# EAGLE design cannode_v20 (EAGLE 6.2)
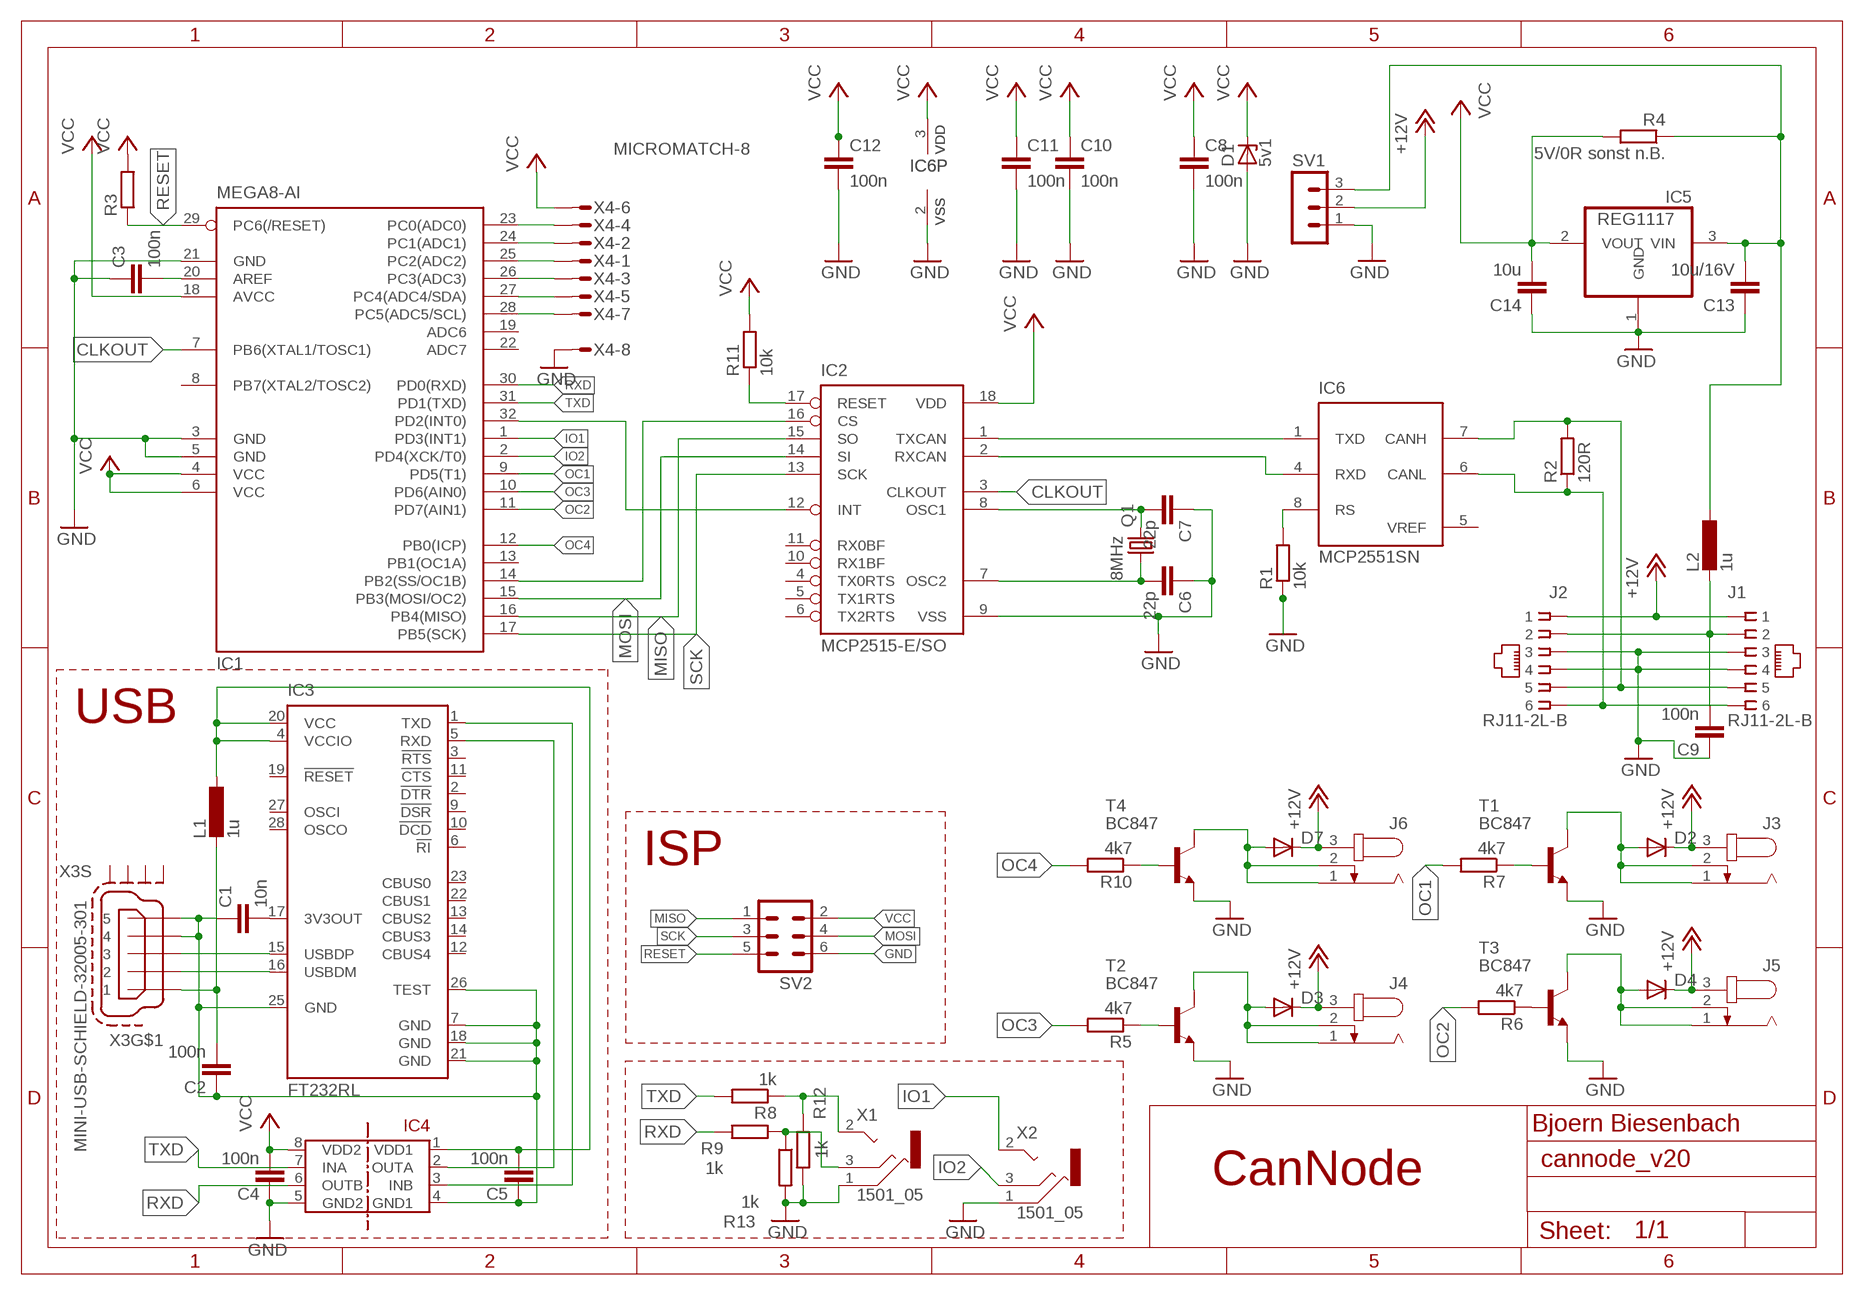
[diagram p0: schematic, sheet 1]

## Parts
C1  10n  C0805  [0805]
C2  100n  C0805  [0805]
C3  100n  C0805  [0805]
C4  100n  C0805  [0805]
C5  100n  C0805  [0805]
C6  22p  C0805  [0805]
C7  22p  C0805  [0805]
C8  100n  C0805  [0805]
C9  100n  C0805  [0805]
C10  100n  C0805  [0805]
C11  100n  C0805  [0805]
C12  100n  C0805  [0805]
C13  10u/16V  C0805  [0805]
C14  10u  C0805  [0805]
D1  5v1  ZENER-DIODESOD80C  [SOD80C]
D2  DIODE-MINIMELF  [MINIMELF]
D3  DIODE-MINIMELF  [MINIMELF]
D4  DIODE-MINIMELF  [MINIMELF]
D7  DIODE-MINIMELF  [MINIMELF]
IC1  MEGA8-AI  [TQFP32-08]
IC2  MCP2515-E/SO  [SO18L]
IC3  FT232RL  [SSOP28]
IC4  ADUM1201  [SO8]
IC5  REG1117  [SOT223]
IC6  MCP2551SN  [SO-08]
J1  RJ11-2L-B  [RJ11-NO_SHIELD]
J2  RJ11-2L-B  [RJ11-NO_SHIELD]
J3  JACK-PLUG0  [SPC4077]
J4  JACK-PLUG0  [SPC4077]
J5  JACK-PLUG0  [SPC4077]
J6  JACK-PLUG0  [SPC4077]
L1  1u  L0805  [0805]
L2  1u  L0805  [0805]
Q1  8MHz  CRYSTALHC49U70  [HC49U70]
R1  10k  R0805  [0805]
R2  120R  R0805  [0805]
R3  R0805  [0805]
R4  5V/0R sonst n.B.  R0805  [0805]
R5  4k7  R0805  [0805]
R6  4k7  R0805  [0805]
R7  4k7  R0805  [0805]
R8  1k  R0805  [0805]
R9  1k  R0805  [0805]
R10  4k7  R0805  [0805]
R11  10k  R0805  [0805]
R12  1k  R0805  [0805]
R13  1k  R0805  [0805]
SV1  MA03-1  [MA03-1]
SV2  MA03-2  [MA03-2]
T1  BC847  [SOT23]
T2  BC847  [SOT23]
T3  BC847  [SOT23]
T4  BC847  [SOT23]
X1  1501_05  [1501_05]
X2  1501_05  [1501_05]
X3  MINI-USB-SCHIELD-32005-301  [32005-301]
X4  MICROMATCH-8  [MICROMATCH-8]

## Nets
+12V: D2.C D3.C D4.C D7.C J1.1 J2.1 J3.3 J4.3 J5.3 J6.3 SV1.2
CLKOUT: IC1.7(PB6(XTAL1/TOSC1)) IC2.3(CLKOUT)
GND: C3.1 C4.1 C6.1 C7.1 C8.2 C9.1 C10.2 C11.2 C12.2 C13.1 C14.1 D1.A IC1.3(GND) IC1.5(GND) IC1.21(GND) IC2.9(VSS) IC4.5(GND2) IC5.1(GND) IC6.2(VSS) J1.3 J1.4 J2.3 J2.4 R1.1 R12.2 R13.2 SV1.1 SV2.6 T1.2(E) T2.2(E) T3.2(E) T4.2(E) X1.1 X2.1 X4.8
GND_USB: C1.1 C2.1 C5.1 IC3.7(GND) IC3.18(GND) IC3.21(GND) IC3.25(GND) IC3.26(TEST) IC4.4(GND1) X3.4 X3.5
IO1: IC1.1(PD3(INT1)) X2.2
IO2: IC1.2(PD4(XCK/T0)) X2.3
MISO: IC1.16(PB4(MISO)) IC2.15(SO) SV2.1
MOSI: IC1.15(PB3(MOSI/OC2)) IC2.14(SI) SV2.4
N$1: C7.2 IC2.8(OSC1) Q1.2
N$2: C6.2 IC2.7(OSC2) Q1.1
N$3: IC2.1(TXCAN) IC6.1(TXD)
N$4: IC2.2(RXCAN) IC6.4(RXD)
N$5: IC6.7(CANH) J1.5 J2.5 R2.2
N$6: IC6.6(CANL) J1.6 J2.6 R2.1
N$7: IC6.8(RS) R1.2
N$8: IC1.14(PB2(SS/OC1B)) IC2.16(CS)
N$9: IC1.32(PD2(INT0)) IC2.12(INT)
N$10: C3.2 IC1.20(AREF)
N$11: IC2.17(RESET) R11.1
N$12: IC3.15(USBDP) X3.3
N$13: IC3.16(USBDM) X3.2
N$14: C5.2 IC3.4(VCCIO) IC3.20(VCC) IC4.1(VDD1) L1.1
N$15: R9.1 R13.1 X1.3
N$16: C9.2 J1.2 J2.2 L2.2
N$17: C2.2 L1.2 X3.1
N$18: C13.2 IC5.3(VIN) L2.1 R4.1 SV1.3
N$20: C1.2 IC3.17(3V3OUT)
N$21: R6.1 T3.1(B)
N$22: D4.A J5.1 J5.2 T3.3(C)
N$24: R5.1 T2.1(B)
N$25: R7.1 T1.1(B)
N$26: IC3.5(RXD) IC4.2(OUTA)
N$27: D2.A J3.1 J3.2 T1.3(C)
N$28: D3.A J4.1 J4.2 T2.3(C)
N$29: IC3.1(TXD) IC4.3(INB)
N$30: R8.1 R12.1 X1.2
N$31: D7.A J6.1 J6.2 T4.3(C)
N$32: IC1.28(PC5(ADC5/SCL)) X4.7
N$33: IC1.27(PC4(ADC4/SDA)) X4.5
N$34: R10.1 T4.1(B)
N$35: IC1.26(PC3(ADC3)) X4.3
N$36: IC1.25(PC2(ADC2)) X4.1
N$37: IC1.24(PC1(ADC1)) X4.2
N$38: IC1.23(PC0(ADC0)) X4.4
OC1: IC1.9(PD5(T1)) R7.2
OC2: IC1.11(PD7(AIN1)) R6.2
OC3: IC1.10(PD6(AIN0)) R5.2
OC4: IC1.12(PB0(ICP)) R10.2
RESET: IC1.29(PC6(/RESET)) R3.1 SV2.5
RXD: IC1.30(PD0(RXD)) IC4.6(OUTB) R9.2
SCK: IC1.17(PB5(SCK)) IC2.13(SCK) SV2.3
TXD: IC1.31(PD1(TXD)) IC4.7(INA) R8.2
VCC: C4.2 C8.1 C10.1 C11.1 C12.1 C14.2 D1.C IC1.4(VCC) IC1.6(VCC) IC1.18(AVCC) IC2.18(VDD) IC4.8(VDD2) IC5.2(VOUT) IC6.3(VDD) R3.2 R4.2 R11.2 SV2.2 X4.6
Unconnected: IC1.8(PB7(XTAL2/TOSC2)) IC1.13(PB1(OC1A)) IC1.19(ADC6) IC1.22(ADC7) IC2.4(TX0RTS) IC2.5(TX1RTS) IC2.6(TX2RTS) IC2.10(RX1BF) IC2.11(RX0BF) IC3.2(!DTR) IC3.3(!RTS) IC3.6(!RI) IC3.9(!DSR) IC3.10(!DCD) IC3.11(!CTS) IC3.12(CBUS4) IC3.13(CBUS2) IC3.14(CBUS3) IC3.19(!RESET) IC3.22(CBUS1) IC3.23(CBUS0) IC3.27(OSCI) IC3.28(OSCO) X3.M1(S:S1) X3.M2(S:S2) X3.M3(S:S3) X3.M4(S:S4)

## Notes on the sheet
- USB
- ISP
- Bjoern Biesenbach
- CanNode

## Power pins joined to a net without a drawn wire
VREF: IC6.5(VREF)

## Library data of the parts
C1-C14 = R_C_0805:C0805
D1 = diode:ZENER-DIODE: Z-Diode
D2-D4 D7 = diode:DIODE-: DIODE
IC1 = atmel:MEGA8: MICROCONTROLLER 8 Kbytes FLASH, 1 kbytes SRAM, 512 bytes EEPROM, USART, 6-channel 10 bit ADC, 2-channel 8 bit ADC Pin compatible with Atmega48, ATMega88, ATMega168 Source: avr.lbr; MPN: ATMEGA8-16AU; OC_FARNELL: 9171371; OC_NEWARK: 73M8863
IC2 = mcp2515:MCP2515
IC3 = ftdichip:FT232R: Source: http://www.ftdichip.com/Documents/DataSheets/DS_FT232R_v104.pdf; MPN: FT232RL; OC_FARNELL: 1146032; OC_NEWARK: 91K9918
IC4 = Bus-isolators:ADUM1201
IC5 = burr-brown:REG1117: 800mA and 1A Low Dropout (LDO) Positive Regulator 1.8V, 2.5V, 2.85V, 3.3V, 5V, and Adj; MPN: REG1117; OC_FARNELL: 1097566; OC_NEWARK: 14P6981
IC6 = microchip_can:MCP2551: High Speed CAN tranceiver
J1 J2 = con-tycoelectronics:RJ11: CORCOM Modular RJ Jacks No Shield Source: www.tycoelectronics.com .. ENG_DS_1654001_1099_RJ_L_0507.pdf; MF: TYCO ELECTRONICS; MPN: RJ11-2L-B; OC_FARNELL: unknown; OC_NEWARK: 83F4463
J3-J6 = con-jack:JACK-PLUG: DC POWER JACK Power Jack, DC, Right Angle, Through Hole, Rated 5A at 16VDC, PC Terminals Distributor: Farnell (www.Farnell.de) Drawing: 84N1161.pdf / 84N1162.pdf Manufacturer: SPC Technology (www.spctechnology.com) Type: SPC4077 / SPC 4078; OC_FARNELL: unknown; OC_NEWARK: unknown
L1 L2 = R_C_0805:L0805
Q1 = crystal:CRYSTAL: CRYSTAL; OC_FARNELL: unknown; OC_NEWARK: unknown
R1-R13 = R_C_0805:R0805
SV1 = con-lstb:MA03-1: PIN HEADER; OC_FARNELL: unknown; OC_NEWARK: unknown
SV2 = con-lstb:MA03-2: PIN HEADER; OC_FARNELL: unknown; OC_NEWARK: unknown
T1-T4 = transistor:BC847: NPN TRANSISTOR
X1 X2 = con-lumberg:1501_0*: Jack connectors according to JISC 6560, 2.5 mm Klinkensteckverbinder nach JISC 6560, 2,5 mm Source: http://www.lumberg.com/Produkte/PDFs/1501_05.pdfedit 1501_03 http://www.lumberg.com/Produkte/PDFs/1501_06.pdf; OC_FARNELL: 1216978; OC_NEWARK: unknown
X3 = con-cypressindustries:MINI-USB-SCHIELD-: MINI USB-B Conector Source: www.cypressindustries.com; OC_FARNELL: unknown; OC_NEWARK: unknown
X4 = con-amp-micromatch:MICROMATCH-8: MicroMaTch 8 7-215464-8 / 0-215464-8 Drawing Number C-215464 DDEController.pdf; MF: FARNELL; MPN: 7-215464-8; OC_FARNELL: 3784642; OC_NEWARK: 26H0301

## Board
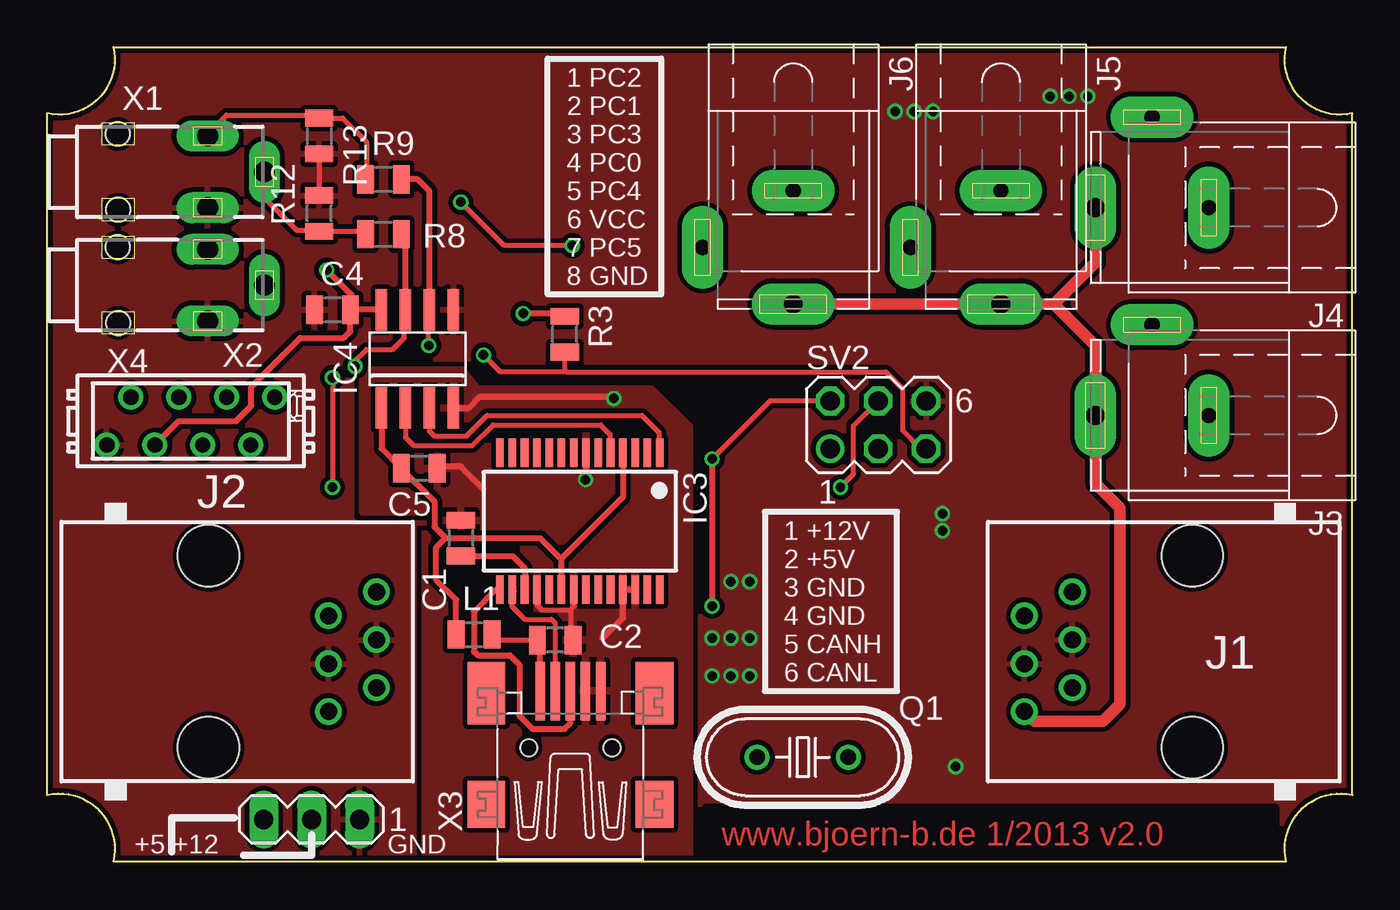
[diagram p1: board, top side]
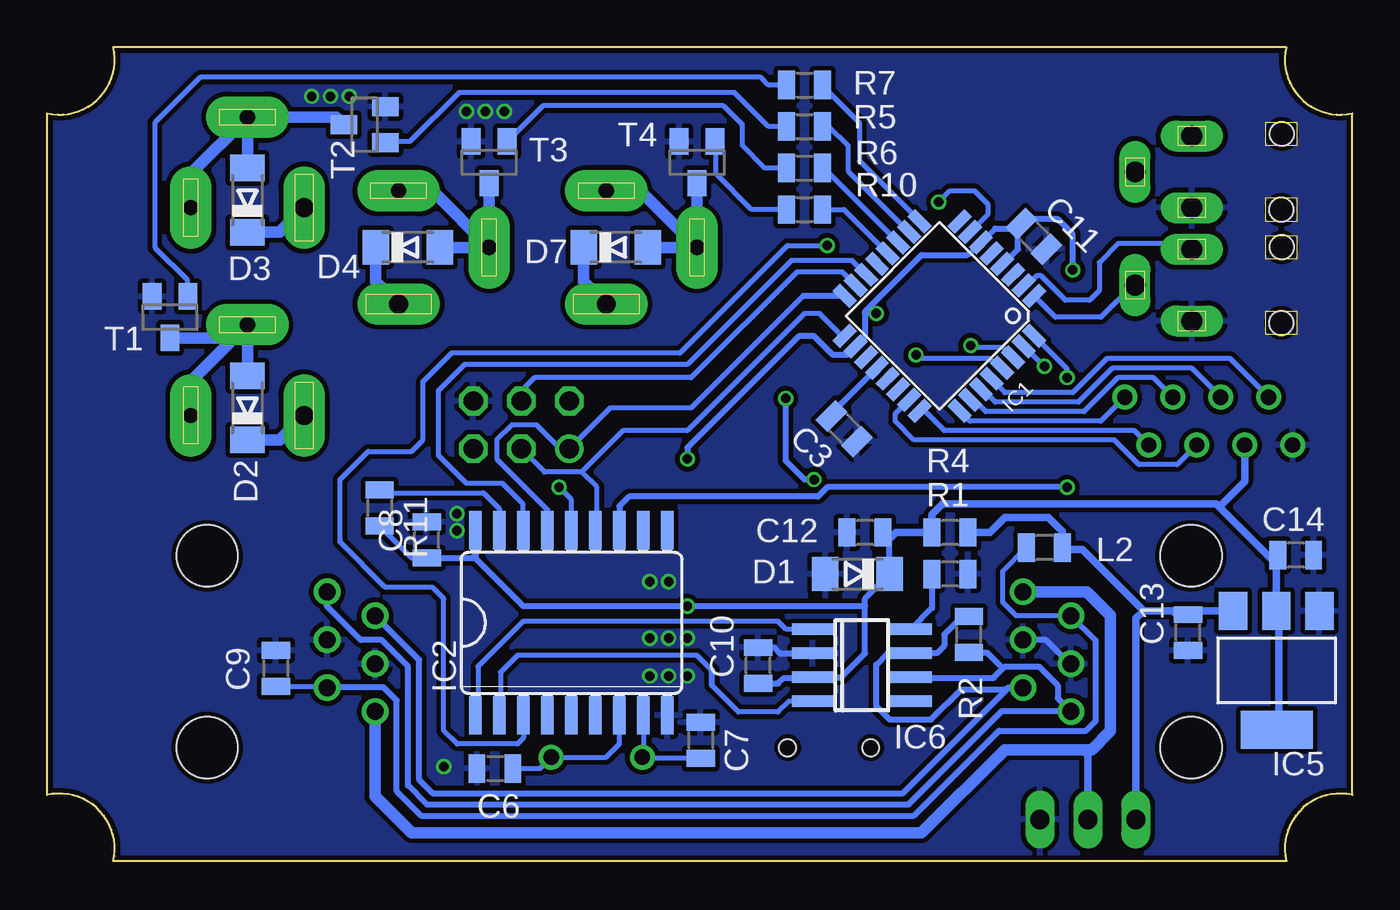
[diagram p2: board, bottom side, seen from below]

Size 69.1 x 43.1 mm. Coordinates in mm from the lower left corner, seen from the top.
Outline: 3.5,0 65.6,0 arc-116 69.1,3.5 69.1,39.6 arc-116 65.6,43.1 3.5,43.1 arc-116 0,39.6 0,3.5 arc-116 3.5,0
Copper layers (1*16): Top 0.035mm / dielectric 1.5mm / Bottom 0.035mm
Design rules: minimum track width 6mil, minimum drill 12mil, track to track 6mil, track to pad 6mil, pad to pad 6mil, via to via 6mil, smd to smd 0mil, copper to edge 10mil, drill to drill 10mil, minimum pad ring 10mil, minimum via ring 6mil, stop-mask expansion 2mil, vias tented up to drill 100mil, thermal gap 10mil
tRestrict: area 34.9,0 to 65,2.8

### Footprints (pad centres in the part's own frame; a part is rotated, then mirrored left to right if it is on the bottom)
0805 = smd 0.894 x 1.5: 1 -0.95,0; 2 0.95,0
SOD80C = smd 1.4 x 1.8: A 1.7,0; C -1.7,0
MINIMELF = smd 1.4 x 1.8: A 1.7,0; C -1.7,0
TQFP32-08 = smd 1.27 x 0.559: 1 -4.293,2.8; 2 -4.293,2; 3 -4.293,1.2; 4 -4.293,0.4; 5 -4.293,-0.4; 6 -4.293,-1.2; 7 -4.293,-2; 8 -4.293,-2.8; 17 4.293,-2.8; 18 4.293,-2; 19 4.293,-1.2; 20 4.293,-0.4; 21 4.293,0.4; 22 4.293,1.2; 23 4.293,2; 24 4.293,2.8 | smd 0.559 x 1.27: 9 -2.8,-4.293; 10 -2,-4.293; 11 -1.2,-4.293; 12 -0.4,-4.293; 13 0.4,-4.293; 14 1.2,-4.293; 15 2,-4.293; 16 2.8,-4.293; 25 2.8,4.293; 26 2,4.293; 27 1.2,4.293; 28 0.4,4.293; 29 -0.4,4.293; 30 -1.2,4.293; 31 -2,4.293; 32 -2.8,4.293
SO18L = smd 0.66 x 2.032: 1 -5.08,-4.902; 2 -3.81,-4.902; 3 -2.54,-4.902; 4 -1.27,-4.902; 5 0,-4.902; 6 1.27,-4.902; 7 2.54,-4.902; 8 3.81,-4.902; 9 5.08,-4.902; 10 5.08,4.902; 11 3.81,4.902; 12 2.54,4.902; 13 1.27,4.902; 14 0,4.902; 15 -1.27,4.902; 16 -2.54,4.902; 17 -3.81,4.902; 18 -5.08,4.902
SSOP28 = smd 0.4 x 1.5: 1 -4.225,-3.625; 2 -3.575,-3.625; 3 -2.925,-3.625; 4 -2.275,-3.625; 5 -1.625,-3.625; 6 -0.975,-3.625; 7 -0.325,-3.625; 8 0.325,-3.625; 9 0.975,-3.625; 10 1.625,-3.625; 11 2.275,-3.625; 12 2.925,-3.625; 13 3.575,-3.625; 14 4.225,-3.625; 15 4.225,3.625; 16 3.575,3.625; 17 2.925,3.625; 18 2.275,3.625; 19 1.625,3.625; 20 0.975,3.625; 21 0.325,3.625; 22 -0.325,3.625; 23 -0.975,3.625; 24 -1.625,3.625; 25 -2.275,3.625; 26 -2.925,3.625; 27 -3.575,3.625; 28 -4.225,3.625
SO8 = smd 0.6 x 2.2: 1 -1.905,-2.6; 2 -0.635,-2.6; 3 0.635,-2.6; 4 1.905,-2.6; 5 1.905,2.6; 6 0.635,2.6; 7 -0.635,2.6; 8 -1.905,2.6
SOT223 = smd 1.499 x 2.007: 1 -2.261,-3.15; 2 0.025,-3.15; 3 2.311,-3.15 | smd 3.81 x 2.007: 4 0,3.15
SO-08 = smd 0.6 x 2.2: 1 -1.905,-2.6; 2 -0.635,-2.6; 3 0.635,-2.6; 4 1.905,-2.6; 5 1.905,2.6; 6 0.635,2.6; 7 -0.635,2.6; 8 -1.905,2.6
RJ11-NO_SHIELD = drill 0.9 pad 1.4: 1 -3.175,8.89; 2 -1.905,6.35; 3 -0.635,8.89; 4 0.635,6.35; 5 1.905,8.89; 6 3.175,6.35 | hole 3.251: -5.08,0; 5.08,0
SPC4077 = drill 0.8 pad 2.184 long: 1 -3,0; 2 0,-4.8 | drill 1 pad 2.184 long: 3 3,0
HC49U70 = drill 0.813: 1 -2.413,0; 2 2.413,0
MA03-1 = drill 1.016 long: 1 -2.54,0; 2 0,0; 3 2.54,0
MA03-2 = drill 1.016: 1 -2.54,-1.27 | drill 1.016 octagon: 2 -2.54,1.27; 3 0,-1.27; 4 0,1.27; 5 2.54,-1.27; 6 2.54,1.27
SOT23 = smd 1 x 1.4: 1 -0.95,-1.1; 2 0.95,-1.1; 3 0,1.1
1501_05 = drill 1.1 pad 1.4 long: 1 -1.9,-8.5; 2 0,-11.5; 3 1.9,-8.5 | hole 1.27: -2.007,-3.759; 2.007,-3.734
32005-301 = smd 3.1 x 0.5: 1 3,1.6; 2 3,0.8; 3 3,0; 4 3,-0.8; 5 3,-1.6 | smd 2.5 x 2: M1 -3,-4.45; M2 -3,4.45 | smd 3.3 x 2: M3 2.9,4.45; M4 2.9,-4.45 | hole 0.9: 0,2.2; 0,-2.2
MICROMATCH-8 = drill 0.813: 1 4.445,1.27; 2 3.175,-1.27; 3 1.905,1.27; 4 0.635,-1.27; 5 -0.635,1.27; 6 -1.905,-1.27; 7 -3.175,1.27; 8 -4.445,-1.27

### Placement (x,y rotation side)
C1  21.9,17.1 270 top
C2  26.9,11.7 180 top
C3  26.9,22.9 135 bottom
C4  15.1,29.2 0 top
C5  19.7,20.8 180 top
C6  45.4,4.9 0 bottom
C7  34.5,6.4 270 bottom
C8  49,17 90 bottom
C9  57,10.2 270 bottom
C10  31.46,10.35 90 bottom
C11  16.86,33.08 315 bottom
C12  25.8,17.4 180 bottom
C13  8.7,12.1 90 bottom
C14  3,16.2 180 bottom
D1  26.2,15.2 180 bottom
D2  58.5,24 90 bottom
D3  58.5,35 90 bottom
D4  50,32.5 0 bottom
D7  39,32.5 0 bottom
IC1  21.85,28.87 225 bottom
IC2  41.34,12.62 0 bottom
IC3  28.2,18 180 top
IC4  19.6,26.6 0 top
IC5  4,10.1 180 bottom
IC6  25.97,10.37 270 bottom
J1  60.63,11.09 90 top
J2  8.54,11.09 270 top
J3  58.5,23.6 180 top
J4  58.5,34.6 180 top
J5  50.5,32.5 270 top
J6  39.5,32.5 270 top
L1  22.6,12 0 top
L2  16.3,16.6 180 bottom
Q1  40,5.5 180 top
R1  21.3,15.2 180 bottom
R2  20.3,12 90 bottom
R3  27.4,27.9 90 top
R4  21.3,17.4 180 bottom
R5  29,38.9 0 bottom
R6  29,36.7 0 bottom
R7  29,41.1 0 bottom
R8  17.8,33.2 0 top
R9  17.8,36.1 0 top
R10  29,34.5 0 bottom
R11  51.5,18.7 270 bottom
R12  14.4,34.3 90 top
R13  14.4,38.4 270 top
SV1  14,2.2 180 top
SV2  44,23.1 0 top
T1  62.6,28.8 180 bottom
T2  52.3,39 90 bottom
T3  45.7,37 180 bottom
T4  34.7,37 180 bottom
X1  0,36.5 90 top
X2  0,30.5 90 top
X3  27.7,6 90 top
X4  7.6,23.3 0 top

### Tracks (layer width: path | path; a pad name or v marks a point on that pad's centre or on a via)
+12V
  Top 0.61: J1.1 52.26,7.4 55.9,7.4 56.8,8.3 56.8,18.7 55.5,20 J3.3 55.5,27.3 53.3,29.5 | 53.3,29.5 J5.3 J6.3 | J4.3 55.5,31.7 53.3,29.5
  Bottom 0.4: SV1.2 14,5.6 14.3,5.9
  Bottom 0.61: J2.1 14.06,14.27 12.8,13 12.8,6.9 13.8,5.9 14.3,5.9 18.4,5.9 22.8,1.5 49.8,1.5 51.74,3.44 J1.1 | J3.3 56.8,22.3 D2.C | D3.C 56.8,33.3 J4.3 | D4.C 51.7,30.7 J5.3 | D7.C 40.7,30.7 J6.3
CLKOUT  (via drill 0.5)
  Top 0.254: v27.8,32.6 24.2,32.6 v21.9,34.9
  Bottom 0.254: IC1.7 19.3,34.25 19.3,34.8 20,35.5 21.3,35.5 v21.9,34.9 | v27.8,32.6 29.9,32.6 35.6,26.9 47.7,26.9 49.2,25.4 49.2,22.3 49.8,21.7 52.1,21.7 53.6,20.2 53.6,16.9 51.2,14.5 48.7,14.5 48.1,13.9 48.1,6.9 47.4,6.2 44.2,6.2 43.88,6.52 IC2.3
GND  (via drill 0.5)
  Top 0.254: R13.2 R12.2
  Bottom 0.305: C10.2 30.6,11.3 30.3,11 IC6.2 | J2.4 14.96,10.46 16.23,11.72 J2.3
  other vias: 44.9,39.7 45.9,39.7 46.9,39.7 53.1,40.5 54.1,40.5 55.1,40.5 47.4,18.4 37.2,11.8 36.2,11.8 35.2,11.8 35.2,9.8 36.2,9.8 37.2,9.8 48.1,5 47.4,17.5 37.2,14.8 36.2,14.8
  pour Bottom (isolate 0.254): 0,0 69,0 69,43 69,43.5 0,43.5
  pour Top (isolate 0.254, rank 2): 0,0 69.5,0 69.5,43 69.5,43.5 0,43.5
GND_USB  (via drill 0.5)
  Top 0.254: IC3.18 25.93,13.57 26.2,13.3 27.7,13.3 | 27.7,13.3 27.9,13.5 27.9,14.35 IC3.21 | 27.7,13.3 27.7,11.95 C2.1
  Top 0.305: IC3.26 IC3.25 30.5,14.35 30.5,12.9 29.4,11.8 | IC3.7 28.52,20.38 28.6,20.3 | IC4.4 22.3,24 22.9,24.6 29.9,24.6 v30,24.5 | 23.1,19.7 21.9,20.9 20.9,20.9 20.7,20.7 20.6,20.7
  Bottom 0.305: v30,24.5 30,21.2 29,20.2 v28.5,20.2
  pour Top (isolate 0.254): 16.7,26 22,26 22.8,25 32,25 34,23 34,0 20,0 20,18.5 16.7,18.5
IO1
  Bottom 0.254: X2.2 11.6,30.5 13.3,28.8 15.71,28.8 IC1.1
IO2
  Bottom 0.254: X2.3 8.8,32.7 12.4,32.7 13.4,31.7 13.4,30.2 13.9,29.7 15.2,29.7 16.5,31 16.7,31 17.1,30.6 | 17.1,30.6 17.21,30.49 IC1.2 | 17.1,30.6 17.2,30.6
MISO
  Bottom 0.254: 29.07,29.93 35,24 39.29,24 SV2.1 41.93,21.83 43.2,23.1 44.5,23.1 45.3,22.3 45.3,21.3 42.6,18.6 42.6,17.53
  Bottom 0.305: IC1.16 29.07,29.93 | 42.6,17.53 IC2.15
MOSI  (via drill 0.5)
  Top 0.254: v42,19.8 42.7,20.5 42.7,23.07 SV2.4
  Bottom 0.254: IC1.15 27,31.2 29.4,31.2 35,25.6 43.3,25.6 44,24.9 SV2.4 | IC2.14 41.34,19.14 v42,19.8
  Bottom 0.305: IC1.15
N$1
  Bottom 0.254: IC2.8 37.53,5.56 Q1.2 37.54,5.45 C7.2
N$2
  Bottom 0.254: C6.2 43.01,4.9 Q1.1 39.5,5.5 38.8,6.2 IC2.7
N$3
  Bottom 0.254: IC6.1 29.98,12.28 30.4,12.7 43.9,12.7 46.3,10.3 46.3,7.84
  Bottom 0.305: 46.3,7.84 IC2.1
N$4
  Bottom 0.254: IC6.4 29.84,8.46 30.4,7.9 32.5,7.9 33.9,9.3 | 33.9,10.1 34.7,10.9 44.2,10.9 45.1,10 45.1,7.77
  Bottom 0.305: 33.9,9.3 33.9,10.1 | 45.1,7.77 IC2.2
N$5
  Bottom 0.305: R2.2 20.65,12.95 21.6,12 21.6,11.4 22,11 IC6.7 24.6,11 25.2,10.4 25.2,8.2 24.5,7.5 22.3,7.5 20.7,9.1 18.4,9.1 18.35,9.05 | J1.5 49.4,10.65 49.4,4.3 48.7,3.6 23.8,3.6 18.35,9.05 | J2.5 18.21,9.19 18.35,9.05
N$6
  Bottom 0.305: IC6.6 23.4,9.7 19,9.7 18.5,10.2 | 18.5,10.2 18.4,10.3 16.6,10.3 15.6,9.3 15.6,8.62 J2.6 18.59,7.92 23.5,3 49,3 50,4 50,10.3 51.4,11.7 52.5,11.7 54.3,13.5 54.3,14.24 J1.6 | R2.1 19.35,11.05 18.5,10.2
N$7
  Bottom 0.305: R1.2 22.25,13.39 IC6.8
N$8
  Bottom 0.254: 25.76,31.06 26.5,31.8 29.7,31.8 35.2,26.3 47,26.3 48.4,24.9 48.4,21.5 46.9,20 45,20 43.9,18.9 43.9,17.54
  Bottom 0.305: IC1.14 25.76,31.06 | 43.9,17.54 IC2.16
N$9  (via drill 0.5)
  Top 0.254: v15.1,25.6 v15.1,19.8
  Bottom 0.254: IC1.32 15.1,26.08 v15.1,25.6
  Bottom 0.305: IC2.12 38.8,18.8 38.3,19.3 28.3,19.3 27.8,19.8 v15.1,19.8
N$10
  Bottom 0.305: C3.2 27.57,23.71 IC1.20
N$11
  Bottom 0.254: IC2.17 45.15,18.65 46,19.5 51.35,19.5 R11.1
N$12
  Top 0.305: IC3.15 24,14.35 23.75,14.35 22.6,13.2 22.6,11.1 22.8,10.9 24.5,10.9 25,10.4 25,7.7 25.7,7 27.4,7 27.7,7.3 X3.3
N$13
  Top 0.254: X3.2 26.9,12.3 26.9,12.5 26.9,12.6 26.7,12.8 25.3,12.8 24.62,13.47 IC3.16
  Top 0.305: 24.7,14.3 IC3.16
N$14
  Top 0.305: L1.1 21.65,13.85 20.6,14.9 20.6,16.6 21.1,17.1 | 21.1,17.1 26.1,17.1 27.2,16 | 27.2,16 27.2,14.4 IC3.20 | IC4.1 17.7,21.86 C5.2 20.5,19.05 20.5,17.7 21.1,17.1 | IC3.4 30.48,19.27 27.2,16
N$15
  Top 0.254: X1.3 8.5,38.5 9.5,39.5 14.25,39.5 R13.1 15.65,39.35 16.9,38.1 16.9,36.15 R9.1
N$16
  Bottom 0.254: J1.2 54.34,9.25 C9.2 57,9.2 56.95,9.15 | J2.2 17.8,12.99 18.5,13.7 18.5,15.35 L2.2
  Bottom 0.305: J2.2 13.6,11.71 13.6,7.4 14.1,6.9 18.7,6.9 23.2,2.4 49.3,2.4 50.6,3.7 50.6,8.5 51.3,9.2 54.27,9.2 J1.2 | 56.91,9.19 56.95,9.15 57,9.1
N$17
  Top 0.254: 23.75,11.8 23.85,11.7 C2.2
  Top 0.305: X3.1 26.1,11.65 C2.2 | 23.75,11.8 L1.2
N$18
  Bottom 0.254: C13.2 9.4,13.05 9.6,13.25
  Bottom 0.4: IC5.3 9.6,13.25 11.05,13.25 | 11.05,13.25 14.3,16.5 15.25,16.5 L2.1 15.35,17.45 16.1,18.2 18.4,18.2 19.2,17.4 R4.1 | SV1.3 11.46,12.84 11.05,13.25
N$20
  Top 0.305: C1.2 24.65,16.15 25.3,15.5 25.3,14.4 IC3.17
N$21
  Bottom 0.254: R6.1 31.1,36.7 32.3,37.9 32.3,39 33.3,40 42.85,40 T3.1
N$22
  Bottom 0.61: J5.1 48.7,35.5 J5.2 | D4.A J5.2 | T3.3 J5.2
N$24
  Bottom 0.254: R5.1 30.9,38.9 32.7,40.7 47.3,40.7 49.9,38.1 51.15,38.1 T2.1
N$25
  Bottom 0.254: R7.1 30.9,41.1 31.3,41.5 61,41.5 63.4,39.1 63.4,32.5 61.7,30.8 61.7,29.95 T1.1
N$26
  Top 0.254: IC4.2 18.96,22.43 19.4,22 22.5,22 23.6,23.1 29.3,23.1 29.8,22.6 29.8,21.65 IC3.5
N$27
  Bottom 0.61: J3.1 61.5,25.4 59.2,27.7 | T1.3 59.2,27.7 | 59.2,27.7 J3.2 D2.A
N$28
  Bottom 0.61: J4.1 61.5,36.4 J4.2 | J4.2 D3.A | J4.2 53.8,39.4 T2.3
N$29
  Top 0.254: IC4.3 20.23,22.77 20.5,22.5 22.2,22.5 23.3,23.6 31.5,23.6 32.4,22.7 32.4,21.65 IC3.1
N$30
  Top 0.254: X1.2 11.5,35.1 13.2,33.4 14.35,33.4 R12.1 16.7,33.35 R8.1
N$31
  Bottom 0.61: J6.1 37.7,35.5 J6.2 | D7.A J6.2 | T4.3 J6.2
N$32
  Bottom 0.254: X4.7 6.46,26.6 13,26.6 14.8,24.8 18.4,24.8 19.1,25.5 IC1.28
N$33
  Bottom 0.254: X4.5 8.49,26.1 12.7,26.1 14.5,24.3 18.9,24.3 19.59,24.99 IC1.27
N$34
  Bottom 0.254: R10.1 31.8,34.5 33.7,36.4 33.7,38.05 T4.1
N$35
  Bottom 0.254: X4.3 10.54,25.6 12.4,25.6 14.2,23.8 19.4,23.8 20.02,24.42 IC1.26
N$36
  Bottom 0.254: X4.1 13.31,23.3 20.24,23.3 IC1.25
N$37
  Bottom 0.254: X4.2 11.54,22.8 21.6,22.8 22.66,23.86 IC1.24
N$38
  Bottom 0.254: X4.4 9.27,21 11.3,21 12.6,22.3 23.2,22.3 24.2,23.3 24.2,23.7 IC1.23
OC1
  Bottom 0.254: R7.2 28.05,41.05 26.1,39.1 26.1,37.08 IC1.9
OC2
  Bottom 0.254: R6.2 27.98,36.7 IC1.11
OC3
  Bottom 0.254: R5.2 27.7,38.9 26.7,37.9 26.7,36.55 IC1.10
OC4
  Bottom 0.254: R10.2 26.91,34.5 IC1.12
RESET  (via drill 0.5)
  Top 0.254: 27.5,25.9 24,25.9 v23.1,26.8 | R3.1 27.4,26 27.5,25.9 | 27.5,25.9 44.4,25.9 45.3,25 45.3,22.8 46.27,21.83 SV2.5
  Bottom 0.254: IC1.29 18.72,26.12 19.2,26.6 22.9,26.6 v23.1,26.8
RXD  (via drill 0.5)
  Top 0.254: v20.2,27.3 20.2,29.16 IC4.6
  Top 0.305: IC4.6 20.23,35.47 19.6,36.1 R9.2
  Bottom 0.254: IC1.30 17.98,26.68 18.5,27.2 20.1,27.2 v20.2,27.3
SCK
  Bottom 0.254: 27.02,27.82 28.2,29 29,29 35.2,22.8 38.6,22.8 40.8,20.6 | 40.8,20.6 42.77,20.6 SV2.3 | 40,17.59 40,19.8 40.8,20.6
  Bottom 0.305: 40,17.59 IC2.13 | IC1.17 27.02,27.82
TXD  (via drill 0.5)
  Top 0.254: v16.3,26.2 16.3,26.5 16.9,27.1 18.3,27.1 18.9,27.7 18.9,29.14 IC4.7
  Top 0.305: IC4.7 18.96,32.98 R8.2
  Bottom 0.254: IC1.31 17.35,27.25 v16.3,26.2
VCC  (via drill 0.5)
  Top 0.254: SV2.2 38.27,24.37 v35.2,21.3
  Top 0.305: 16.1,29.2 C4.2 16.05,28.05 15.7,27.7 13.4,27.7 10.8,25.1 10.8,24.1 10,23.3 6.96,23.3 X4.6 | IC4.8 16.1,29.2 | 16.1,29.2 16.1,30 v14.8,31.3 | v35.2,21.3 v35.2,13.5 | R3.2 27.25,29 v25.2,29
  Bottom 0.254: 19.65,32.75 18.9,33.5 | IC1.6 20.32,32.1 20.4,32.1 | R11.2 49.8,16.05 C8.1 | C14.2 4.5,16.2 4.8,16.5
  Bottom 0.305: C10.1 30.4,9.4 30.1,9.7 28.61,9.7 IC6.3 27.07,9.73 25.8,11 25.8,13.5 | IC1.4 18.48,31.62 17.7,32.4 17.7,33.59 C11.1 | IC1.6 19.65,32.75 | 18.9,33.5 17.79,33.5 C11.1 | C12.1 24.5,17.05 D1.C 25.8,13.9 25.8,13.5 | IC1.18 25.8,27.75 25.8,27.8 | 25.8,29 25.8,29.1 22.8,32.1 20.4,32.1 | IC2.18 46.42,16.2 | 46.42,16.2 46.42,16.02 43.9,13.5 v35.2,13.5 25.8,13.5 | C8.1 46.57,16.05 46.42,16.2 | v14.8,31.3 14.8,33.2 15.6,34 17.29,34 C11.1 | IC1.18 26.75,26.8 27.5,26.8 28.5,27.8 29.3,27.8 35.2,21.9 v35.2,21.3 | v25.2,29 25.8,29 | 25.8,29 25.8,27.8 | 25.8,27.8 26.3,27.3 IC1.18
  Bottom 0.4: 7.05,18.75 4.8,16.5 4.03,15.72 IC5.2 3.9,13.12 3.9,6.8 3.8,6.7 | 7.05,18.75 7.2,18.9 21.7,18.9 22.25,18.35 R4.2 24.15,17.4 24.5,17.05 | X4.6 5.7,20.11 7.05,18.75

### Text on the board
Top: www.bjoern-b.de 1/2013 v2.0
tPlace: +5 +12 | GND
tNames: 1 PC2 | 2 PC1 | 3 PC3 | 4 PC0 | 5 PC4 | 6 VCC | 7 PC5 | 8 GND | 1 +12V | 2 +5V | 3 GND | 4 GND | 5 CANH | 6 CANL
